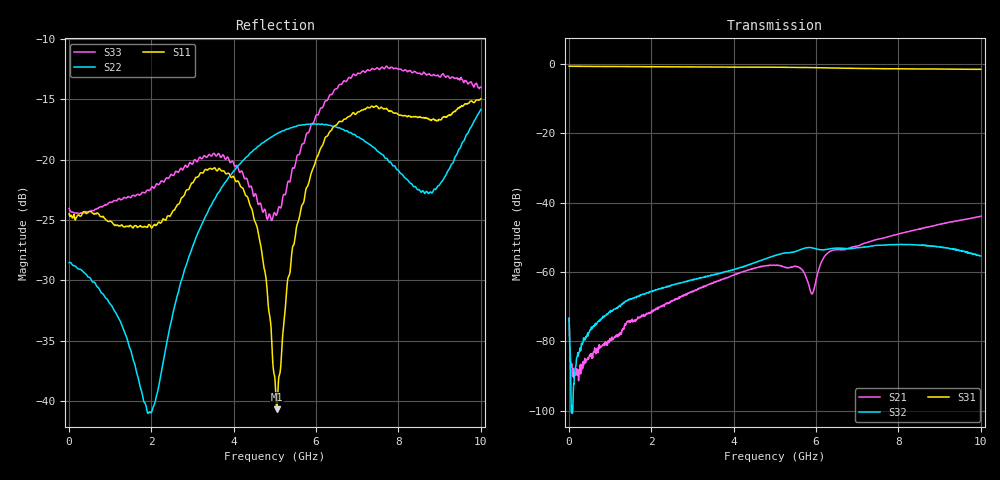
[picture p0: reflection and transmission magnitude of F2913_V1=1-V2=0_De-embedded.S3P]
! 515 Groton Road, Suite 102
! Westford, MA 01886-6024
! Device:  F2913
! Description: High Isolation SP2T RF Switch
! Frequency:  0.050 -  6.000 GHz
! Package:  4x4 mm QFN Plastic Package: 20 pin
! Ports:  3 RF, 3 DC
!  Pin  1  = GND
!  Pin  2  = GND
!  Pin  3  = RF1  =  Port 1
!  Pin  4  = GND
!  Pin  5  = GND
!  Pin  6  = GND
!  Pin  7  = GND
!  Pin  8  = RFC  =  Port 3
!  Pin  9  = GND
!  Pin 10  = GND
!  Pin 11  = GND
!  Pin 12  = GND
!  Pin 13  = RF2  =  Port 2
!  Pin 14  = GND
!  Pin 15  = GND
!  Pin 16  = C2
!  Pin 17  = C1
!  Pin 18  = GND
!  Pin 19  = GND
!  Pin 20  = Vdd
! State:  RF1 Selected
! C1:  +3.3 V (Logic High)
! C2:  0.0 V (Logic Low)
! Voltage:  +3.30  Volts
! Current:  0.082 mA
! Data:  The device was measured on a F2913 evaluation board which has
!  individual transmission lines to the RF pins.  Data was collected
!  using a calibrated network analyzer.  The evaluation board was
!  de-embedded using a AFR (Keysight Technologies).
!  The reference plane is the edge of the package pin.
! Misc:
!  Action Tracker AT0430
!  WorkFront Reference Number 1053824
! Date Measured:  2018-08-23
! Date:  2018-08-24  MJV
! Note:
!  Integrated Device Technology supplies this data as a sample of measured
!  data at the package pin for this product.  Your particular data for this
!  product may vary.
!  Data was taken at 25 degrees C.
!  Integrated Device Technology reserves the right to change this data at anytime.
!Freq_(GHz)  S11M_(dB)  S11P_(deg)  S12M_(dB)  S12P_(deg)  S13M_(dB)  S13P_(deg)
!  S21M_(dB)  S21P_(deg)  S22M_(dB)  S22P_(deg)  S23M_(dB)  S23P_(deg)
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# Hz S dB R 50
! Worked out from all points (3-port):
!   1000 points, 10 MHz to 10 GHz, reference 50 ohm
!   strongest paths, dB at 10 MHz, 2.51 GHz, 5.01 GHz, 7.51 GHz, 10 GHz:
!     S31: -0.7, -0.9, -1.0, -1.4, -1.6
!     S32: -73.4, -63.7, -55.2, -52.2, -55.4
!     S21: -73.3, -68.3, -58.1, -50.5, -43.9
!   lowest |S11| = -40.6 dB at 5.05 GHz (marker M1), VSWR 1.02, Z = 50.1 + j0.927 ohm
!   |S11| at or under -10 dB: start of sweep to end of sweep
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1e7  -24.48 -1.7  -73.36 -46.8  -0.69 -0.3
     -73.31 -47.4  -28.54 -179.7  -73.68 -47.8
     -0.67 -0.3  -73.36 -46.2  -24.05 -1.9
9.3e8  -25.05 -23.1  -80.14 -119.3  -0.78 -14.9
       -80.87 -121.0  -31.54 176.1  -72.01 80.4
       -0.78 -14.9  -72.00 81.4  -23.71 -27.5
1.97e9  -25.42 -18.5  -71.38 -138.0  -0.84 -31.4
        -71.67 -137.5  -40.87 122.6  -65.58 78.6
        -0.84 -31.4  -65.65 78.7  -22.54 -30.4
4.13e9  -21.90 5.5  -60.40 169.1  -0.95 -66.3
        -60.34 169.3  -20.45 87.6  -58.74 78.2
        -0.95 -66.4  -58.86 78.6  -20.93 -21.1
5.01e9  -38.47 64.4  -58.04 139.3  -0.97 -80.9
        -58.07 139.3  -17.95 103.2  -55.23 71.8
        -0.98 -80.8  -55.18 71.7  -24.48 -89.5
5.05e9  -40.64 85.2  -57.93 137.7  -0.97 -81.6
        -57.96 137.4  -17.88 103.9  -55.03 71.2
        -0.98 -81.6  -55.08 71.4  -24.55 -97.3
5.9e9  -20.96 152.2  -66.23 144.1  -1.10 -95.4
       -66.37 145.5  -17.09 117.9  -53.04 51.8
       -1.10 -95.4  -53.03 51.9  -17.02 -149.8
6.27e9  -18.07 149.6  -54.65 164.0  -1.17 -101.3
        -54.65 163.9  -17.13 122.9  -53.42 49.8
        -1.17 -101.3  -53.45 49.7  -15.12 -158.2
8.77e9  -16.71 57.3  -46.87 102.9  -1.48 -139.7
        -46.87 102.6  -22.69 84.9  -52.43 18.4
        -1.48 -139.8  -52.50 18.6  -13.01 -157.2
1e10  -14.98 12.5  -43.96 77.6  -1.58 -161.1
      -43.93 77.4  -15.86 39.7  -55.38 -4.0
      -1.58 -161.2  -55.38 -2.9  -14.03 -159.4
